FUNCTION "FC_GRP_81_R14" : VOID
TITLE =GROUP =81_R14
VERSION : 0.1


VAR_TEMP
  CL : "UDT_CABINET";	//CABINET LOCAL
  CR : "UDT_CABINET";	//CABINET REMOTE
  RelError : BOOL ;	//ERROR RELEASE
  RelErrorCL : BOOL ;	//ERROR RELEASE FROM CABINET LOCAL
  RelErrorCR : BOOL ;	//ERROR RELEASE FROM CABINET REMOTE
  RelControl : BOOL ;	//CONTROL RELEASE
  RelControlCL : BOOL ;	//CONTROL RELEASE FROM CABINET LOCAL
  RelControlCR : BOOL ;	//CONTROL RELEASE FROM CABINET REMOTE
  ErrorConfirm : BOOL ;	//ERROR CONFIRM
  AutoOn : BOOL ;	//AUTOMATIC ON
  AutoOff : BOOL ;	//AUTOMATIC OFF
  RelAuto : BOOL ;	//AUTOMATIC RELEASE
  TempSetpoint : WORD ;
  LAMP_ON : BOOL ;
END_VAR
BEGIN
NETWORK
TITLE =GLOBAL SIGNALS
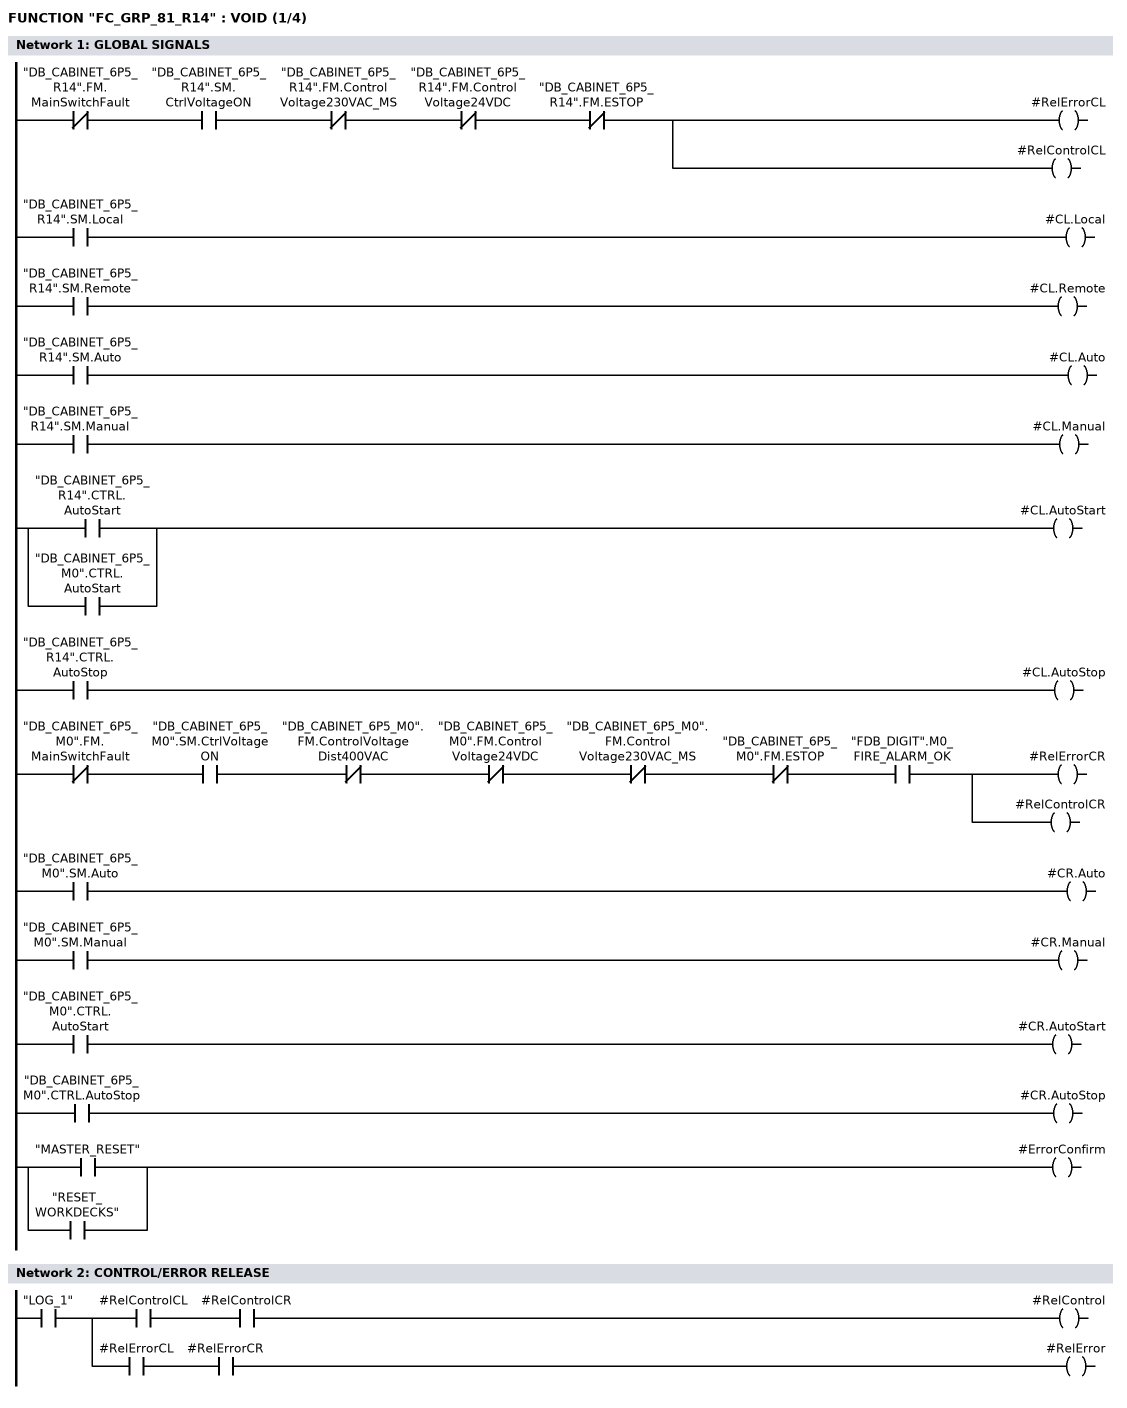
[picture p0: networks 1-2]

      UN    "DB_CABINET_6P5_R14".FM.MainSwitchFault;
      U     "DB_CABINET_6P5_R14".SM.CtrlVoltageON;
      UN    "DB_CABINET_6P5_R14".FM.ControlVoltage230VAC_MS;
      UN    "DB_CABINET_6P5_R14".FM.ControlVoltage24VDC;
      UN    "DB_CABINET_6P5_R14".FM.ESTOP;
      =     #RelErrorCL;
      =     #RelControlCL;

      U     "DB_CABINET_6P5_R14".SM.Local;
      =     #CL.Local;
      U     "DB_CABINET_6P5_R14".SM.Remote;
      =     #CL.Remote;
      U     "DB_CABINET_6P5_R14".SM.Auto;
      =     #CL.Auto;
      U     "DB_CABINET_6P5_R14".SM.Manual;
      =     #CL.Manual;
      U     "DB_CABINET_6P5_R14".CTRL.AutoStart;
      O     "DB_CABINET_6P5_M0".CTRL.AutoStart;
      =     #CL.AutoStart;
      U     "DB_CABINET_6P5_R14".CTRL.AutoStop;
      =     #CL.AutoStop;


      UN    "DB_CABINET_6P5_M0".FM.MainSwitchFault;
      U     "DB_CABINET_6P5_M0".SM.CtrlVoltageON;
      UN    "DB_CABINET_6P5_M0".FM.ControlVoltageDist400VAC;
      UN    "DB_CABINET_6P5_M0".FM.ControlVoltage24VDC;
      UN    "DB_CABINET_6P5_M0".FM.ControlVoltage230VAC_MS;
      UN    "DB_CABINET_6P5_M0".FM.ESTOP;
      U     "FDB_DIGIT".M0_FIRE_ALARM_OK;
      =     #RelErrorCR;
      =     #RelControlCR;

      U     "DB_CABINET_6P5_M0".SM.Auto;
      =     #CR.Auto;
      U     "DB_CABINET_6P5_M0".SM.Manual;
      =     #CR.Manual;
      U     "DB_CABINET_6P5_M0".CTRL.AutoStart;
      =     #CR.AutoStart;
      U     "DB_CABINET_6P5_M0".CTRL.AutoStop;
      =     #CR.AutoStop;


      U     "MASTER_RESET";
      O     "RESET_WORKDECKS";
      =     #ErrorConfirm;

NETWORK
TITLE =CONTROL/ERROR RELEASE

      U     "LOG_1";
      =     L      9.0;
      U     L      9.0;
      U     #RelControlCL;
      U     #RelControlCR;
      =     #RelControl;
      U     L      9.0;
      U     #RelErrorCL;
      U     #RelErrorCR;
      =     #RelError;
NETWORK
TITLE =SUPPLY AIR FAN =81FAN01, CONTROL SIGNALS
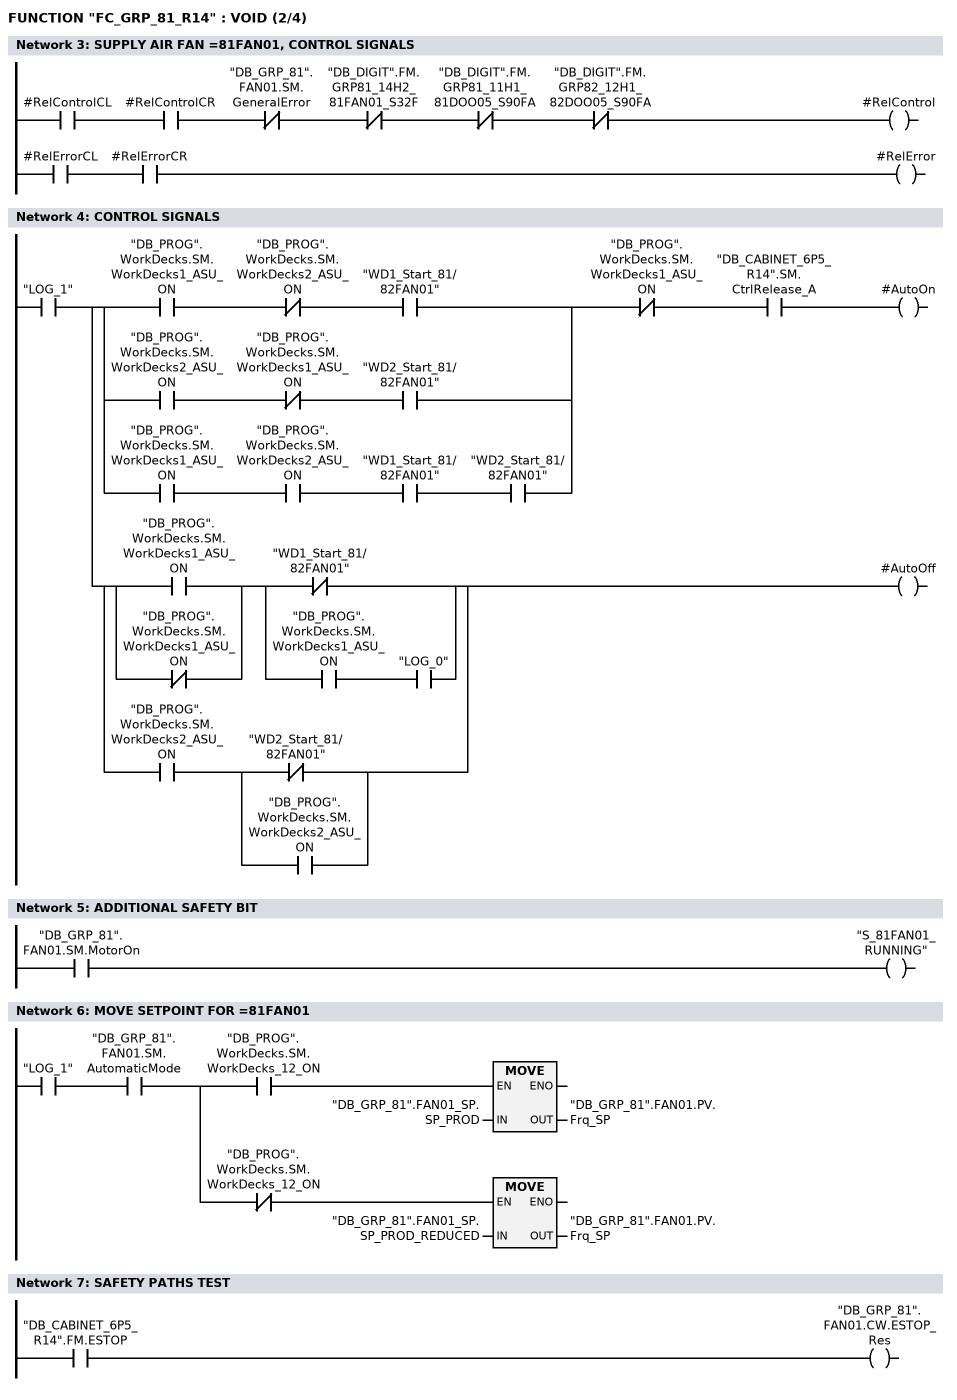
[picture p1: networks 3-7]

      U     #RelControlCL;
      U     #RelControlCR;
      UN    "DB_GRP_81".FAN01.SM.GeneralError;
      UN    "DB_DIGIT".FM.GRP81_14H2_81FAN01_S32F;
//      AN    "6P5_81FAN01+14H2-A85:27"
      UN    "DB_DIGIT".FM.GRP81_11H1_81DOO05_S90FA;
      UN    "DB_DIGIT".FM.GRP82_12H1_82DOO05_S90FA;
      =     #RelControl;

      U     #RelErrorCL;
      U     #RelErrorCR;
      =     #RelError;



NETWORK
TITLE =CONTROL SIGNALS

      U     "LOG_1";
      =     L      9.0;
      U     L      9.0;
      U(    ;
      U     "DB_PROG".WorkDecks.SM.WorkDecks1_ASU_ON;
      UN    "DB_PROG".WorkDecks.SM.WorkDecks2_ASU_ON;
      U     "WD1_Start_81/82FAN01";
      O     ;
      U     "DB_PROG".WorkDecks.SM.WorkDecks2_ASU_ON;
      UN    "DB_PROG".WorkDecks.SM.WorkDecks1_ASU_ON;
      U     "WD2_Start_81/82FAN01";
      O     ;
      U     "DB_PROG".WorkDecks.SM.WorkDecks1_ASU_ON;
      U     "DB_PROG".WorkDecks.SM.WorkDecks2_ASU_ON;
      U     "WD1_Start_81/82FAN01";
      U     "WD2_Start_81/82FAN01";
      )     ;
      UN    "DB_PROG".WorkDecks.SM.WorkDecks1_ASU_ON;
      U     "DB_CABINET_6P5_R14".SM.CtrlRelease_A;
      =     #AutoOn;
      U     L      9.0;
      U(    ;
      U(    ;
      O     "DB_PROG".WorkDecks.SM.WorkDecks1_ASU_ON;
      ON    "DB_PROG".WorkDecks.SM.WorkDecks1_ASU_ON;
      )     ;
      U(    ;
      ON    "WD1_Start_81/82FAN01";
      O     ;
      U     "DB_PROG".WorkDecks.SM.WorkDecks1_ASU_ON;
      U     "LOG_0";
      )     ;
      O     ;
      U     "DB_PROG".WorkDecks.SM.WorkDecks2_ASU_ON;
      U(    ;
      ON    "WD2_Start_81/82FAN01";
      O     "DB_PROG".WorkDecks.SM.WorkDecks2_ASU_ON;
      )     ;
      )     ;
      =     #AutoOff;
NETWORK
TITLE =ADDITIONAL SAFETY BIT

      U     "DB_GRP_81".FAN01.SM.MotorOn;
      =     "S_81FAN01_RUNNING";
NETWORK
TITLE =MOVE SETPOINT FOR =81FAN01

      U     "LOG_1";
      U     "DB_GRP_81".FAN01.SM.AutomaticMode;
      =     L      9.0;
      U     L      9.0;
      U     "DB_PROG".WorkDecks.SM.WorkDecks_12_ON;
      SPBNB _001;
      L     "DB_GRP_81".FAN01_SP.SP_PROD;
      T     "DB_GRP_81".FAN01.PV.Frq_SP;
_001: NOP   0;
      U     L      9.0;
      UN    "DB_PROG".WorkDecks.SM.WorkDecks_12_ON;
      SPBNB _002;
      L     "DB_GRP_81".FAN01_SP.SP_PROD_REDUCED;
      T     "DB_GRP_81".FAN01.PV.Frq_SP;
_002: NOP   0;
NETWORK
TITLE =SAFETY PATHS TEST

      U     "DB_CABINET_6P5_R14".FM.ESTOP;
      =     "DB_GRP_81".FAN01.CW.ESTOP_Res;
NETWORK
TITLE =COAST DOWN ENABLED 81FAN01
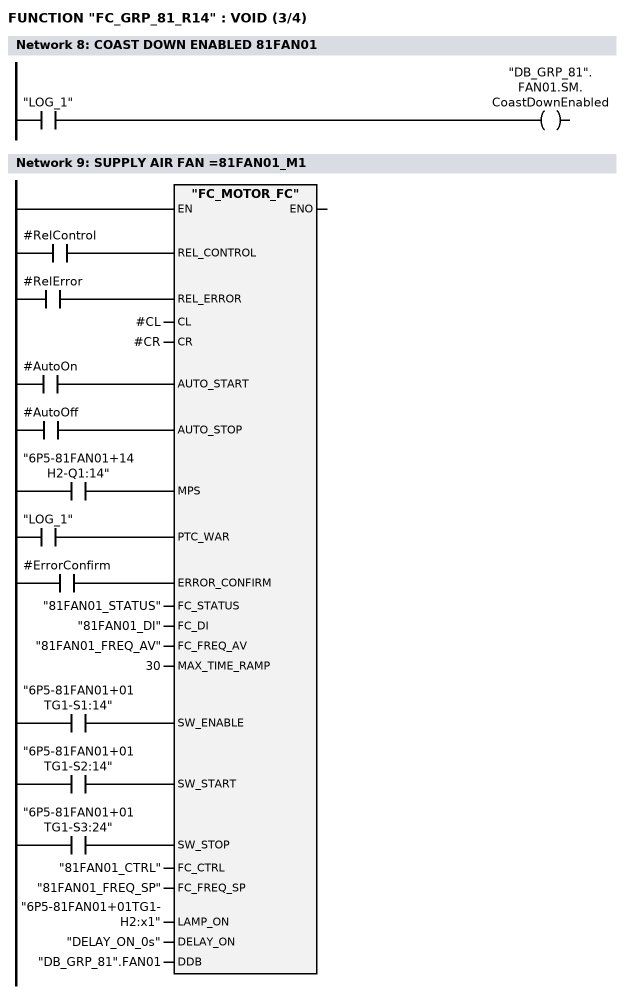
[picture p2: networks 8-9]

      U     "LOG_1";
      =     "DB_GRP_81".FAN01.SM.CoastDownEnabled;
NETWORK
TITLE =SUPPLY AIR FAN =81FAN01_M1

      U     #RelControl;
      =     L      9.0;
      BLD   103;
      U     #RelError;
      =     L      9.1;
      BLD   103;
      U     #AutoOn;
      =     L      9.2;
      BLD   103;
      U     #AutoOff;
      =     L      9.3;
      BLD   103;
      U     "6P5-81FAN01+14H2-Q1:14";
      =     L      9.4;
      BLD   103;
      U     "LOG_1";
      =     L      9.5;
      BLD   103;
      U     #ErrorConfirm;
      =     L      9.6;
      BLD   103;
      U     "6P5-81FAN01+01TG1-S1:14";
      =     L      9.7;
      BLD   103;
      U     "6P5-81FAN01+01TG1-S2:14";
      =     L     10.0;
      BLD   103;
      U     "6P5-81FAN01+01TG1-S3:24";
      =     L     10.1;
      BLD   103;
      CALL "FC_MOTOR_FC" (
           REL_CONTROL              := L      9.0,
           REL_ERROR                := L      9.1,
           CL                       := #CL,
           CR                       := #CR,
           AUTO_START               := L      9.2,
           AUTO_STOP                := L      9.3,
           MPS                      := L      9.4,
           PTC_WAR                  := L      9.5,
           ERROR_CONFIRM            := L      9.6,
           FC_STATUS                := "81FAN01_STATUS",
           FC_DI                    := "81FAN01_DI",
           FC_FREQ_AV               := "81FAN01_FREQ_AV",
           MAX_TIME_RAMP            := 30,
           SW_ENABLE                := L      9.7,
           SW_START                 := L     10.0,
           SW_STOP                  := L     10.1,
           FC_CTRL                  := "81FAN01_CTRL",
           FC_FREQ_SP               := "81FAN01_FREQ_SP",
           LAMP_ON                  := "6P5-81FAN01+01TG1-H2:x1",
           DELAY_ON                 := "DELAY_ON_0s",
           DDB                      := "DB_GRP_81".FAN01);
      NOP   0;
NETWORK
TITLE =PRESSURE SENSOR, =81FAN01_S32F
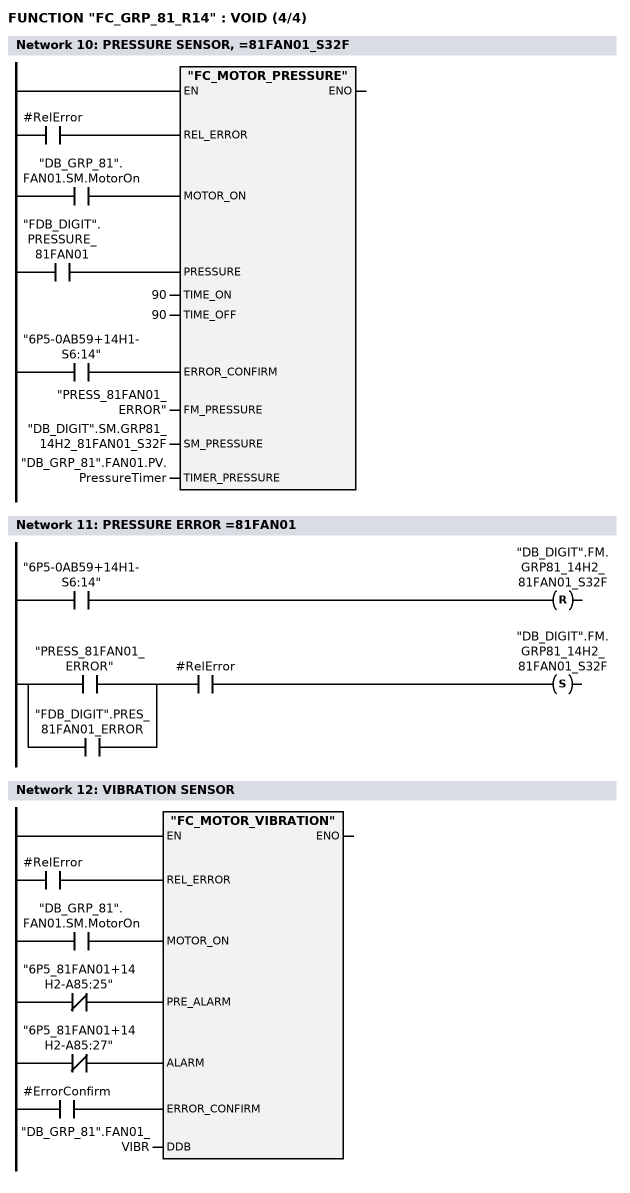
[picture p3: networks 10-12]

      U     #RelError;
      =     L      9.0;
      BLD   103;
      U     "DB_GRP_81".FAN01.SM.MotorOn;
      =     L      9.1;
      BLD   103;
      U     "FDB_DIGIT".PRESSURE_81FAN01;
      =     L      9.2;
      BLD   103;
      U     "6P5-0AB59+14H1-S6:14";
      =     L      9.3;
      BLD   103;
      CALL "FC_MOTOR_PRESSURE" (
           REL_ERROR                := L      9.0,
           MOTOR_ON                 := L      9.1,
           PRESSURE                 := L      9.2,
           TIME_ON                  := 90,
           TIME_OFF                 := 90,
           ERROR_CONFIRM            := L      9.3,
           FM_PRESSURE              := "PRESS_81FAN01_ERROR",
           SM_PRESSURE              := "DB_DIGIT".SM.GRP81_14H2_81FAN01_S32F,
           TIMER_PRESSURE           := "DB_GRP_81".FAN01.PV.PressureTimer);
      NOP   0;
NETWORK
TITLE =PRESSURE ERROR =81FAN01

      U     "6P5-0AB59+14H1-S6:14";
      R     "DB_DIGIT".FM.GRP81_14H2_81FAN01_S32F;
      U(    ;
      O     "PRESS_81FAN01_ERROR";
      O     "FDB_DIGIT".PRES_81FAN01_ERROR;
      )     ;
      U     #RelError;
      S     "DB_DIGIT".FM.GRP81_14H2_81FAN01_S32F;
      NOP   0;
NETWORK
TITLE =VIBRATION SENSOR

      U     #RelError;
      =     L      9.0;
      BLD   103;
      U     "DB_GRP_81".FAN01.SM.MotorOn;
      =     L      9.1;
      BLD   103;
      UN    "6P5_81FAN01+14H2-A85:25";
      =     L      9.2;
      BLD   103;
      UN    "6P5_81FAN01+14H2-A85:27";
      =     L      9.3;
      BLD   103;
      U     #ErrorConfirm;
      =     L      9.4;
      BLD   103;
      CALL "FC_MOTOR_VIBRATION" (
           REL_ERROR                := L      9.0,
           MOTOR_ON                 := L      9.1,
           PRE_ALARM                := L      9.2,
           ALARM                    := L      9.3,
           ERROR_CONFIRM            := L      9.4,
           DDB                      := "DB_GRP_81".FAN01_VIBR);
      NOP   0;
NETWORK
TITLE =END

END_FUNCTION

